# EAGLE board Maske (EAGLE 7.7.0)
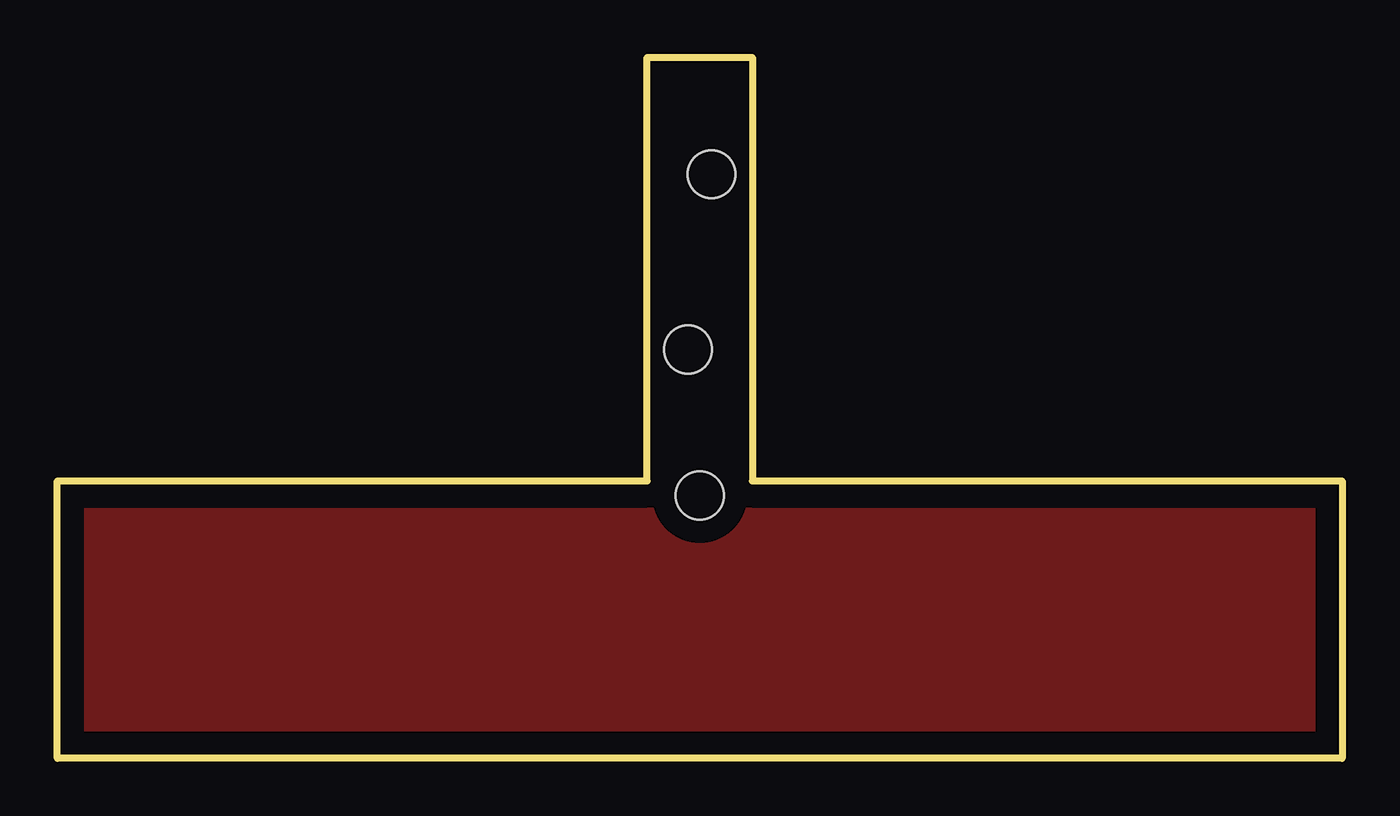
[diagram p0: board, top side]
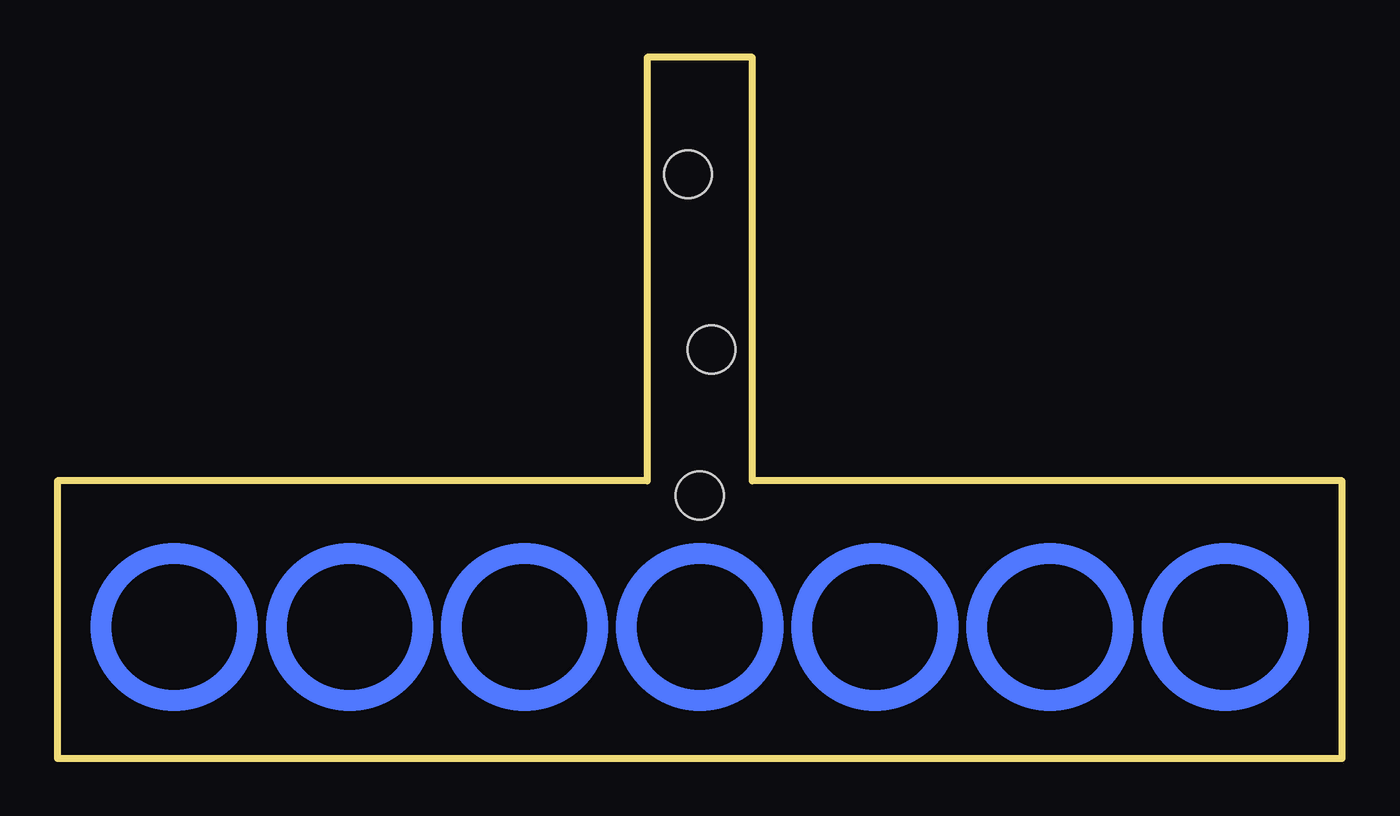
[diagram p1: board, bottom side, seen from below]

Size 55.88 x 30.48 mm. Coordinates in mm from the lower left corner, seen from the top.
Outline: 0,12.06 25.65,12.06 25.65,30.48 30.23,30.48 30.23,12.06 55.88,12.06 55.88,0 0,0 0,12.06
Copper layers (1*16): Top 0.035mm / dielectric 1.5mm / Bottom 0.035mm
Design rules "default": minimum track width 6mil, minimum drill 0.35mm, track to track 6mil, track to pad 6mil, pad to pad 6mil, via to via 6mil, smd to smd 6mil, copper to edge 40mil, drill to drill 6mil, minimum pad ring 10mil, minimum via ring 8mil, stop-mask expansion 4mil, vias tented up to drill 0mil, thermal gap 10mil
Holes 2.08 mm at 27.94,11.43 27.43,17.78 28.45,25.4

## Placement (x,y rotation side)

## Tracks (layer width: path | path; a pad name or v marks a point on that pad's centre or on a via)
X
  pour Top: 0,11.43 0,0 55.88,0 55.88,5.08 55.88,11.43
(copper drawn outside any net)
  shapes: Bottom circle x7

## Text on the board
tStop: MO | DI | MI | DO | FR | SA | SO
tRestrict: MO | DI | MI | DO | FR | SA | SO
